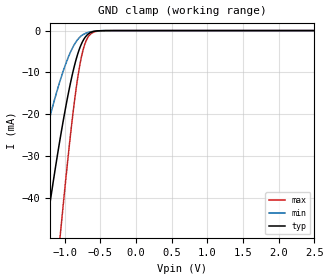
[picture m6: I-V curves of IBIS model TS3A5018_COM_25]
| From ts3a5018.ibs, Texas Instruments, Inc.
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[Model]   TS3A5018_COM_25
Model_type  Terminator
| variable   typ   min   max
C_comp   6.76pF   5.86pF   7.42pF
| C_tri-state   6.76pF   5.86pF   7.42pF
[Temperature Range]   40   100   -40
| Ambient temperature   25   85   -40
[Voltage range]   2.5   2.3   2.7
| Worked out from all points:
|   GND clamp passes 1 mA (typ) near -0.68 V on its own axis
[GND Clamp]
| TS3A5018_COM_25
|   Voltage   I(typ)   I(min)   I(max)
-2.5V     -244.5mA   -152.1mA   -374.1mA
-1.555V   -86.86mA   -48mA      -147.8mA
-1.26V    -47.86mA   -24.4mA    -86.38mA
-1.06V    -25.67mA   -11.86mA   -48.92mA
-1.035V   -23.17mA   -10.52mA   -44.51mA
-960mV    -16.16mA   -6.908mA   -31.78mA
-865mV    -8.658mA   -3.389mA   -17.43mA
-795mV    -4.555mA   -1.73mA    -9.127mA
-735mV    -2.229mA   -910.5uA   -4.286mA
-645mV    -549.5uA   -340.7uA   -993.7uA
-515mV    -45.54uA   -50.44uA   -94.99uA
2.5V      2.125nA    114.1pA    21.18nA
